(* Logix 5000 Controller export Example_PLC; controller Example_PLC 1769-L32E rev 19.11; software revision 19.01; part 2 of 6 *)

ADD_ON_INSTRUCTION AKD_Set_Decel   (* revision 2.1, ExecutePrescan, ExecuteEnableInFalse *)
// Set Drive Deceleration
// Revision note:
// Don't error if Command_Timeout preset is 0
VAR_OUTPUT
   DN : BOOL; {access Read Only, visible}   // Command Successful
   ER : BOOL; {access Read Only, visible}   // Error
END_VAR
VAR_IN_OUT
   Axis : AKD_Axis; {required}
END_VAR
VAR_INPUT
   Decel : DINT; {required}   // Acceleration
END_VAR
VAR
   Response_Bytes : SINT[8];
   OS_LoadStart : BOOL;
   Decel_Internal : DINT;   // Scaled Decel Value for Drive
   Command_Timeout : TIMER := (PRE := 100);   // Timeout Timer
   Command_Message_Type : SINT;   // Command Message Type
   Command_Axis_Number : SINT;   // Command Axis Number
   Response_Message_Type : SINT;   // Response Message Type
   Response_Axis_Number : SINT;   // Response Axis Number
   Command_Bytes : SINT[8];
   Step : SINT;
END_VAR

ROUTINE EnableInFalse   (* ladder *)
// EnableIn_False
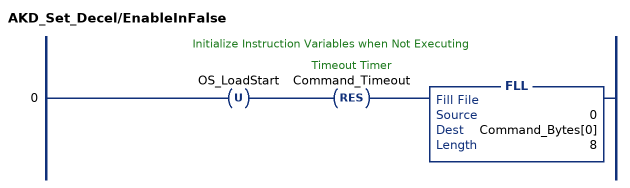
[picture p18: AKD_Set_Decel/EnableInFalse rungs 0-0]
   // Initialize Instruction Variables when Not Executing
   0: OTU(OS_LoadStart)RES(Command_Timeout)FLL(0,Command_Bytes[0],8);
END_ROUTINE

ROUTINE Logic   (* ladder *)
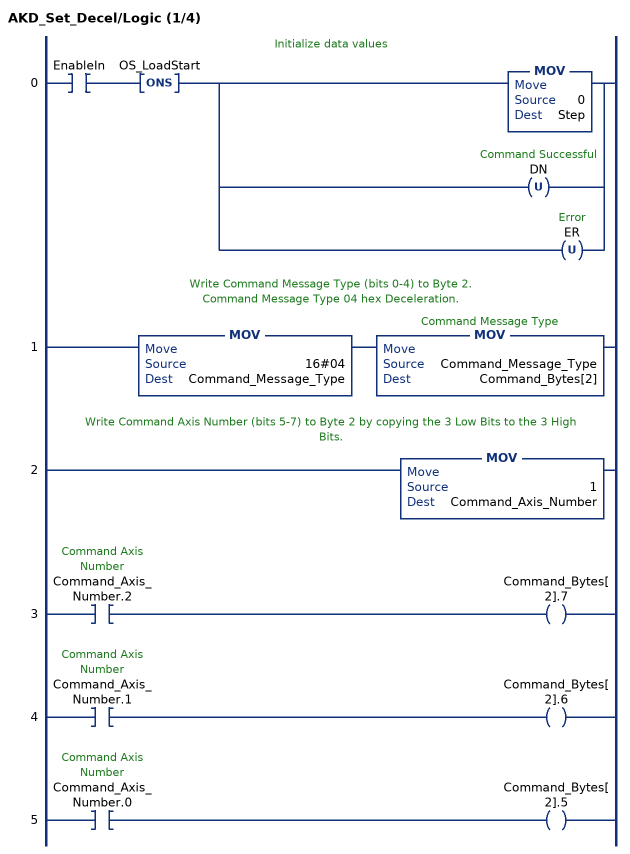
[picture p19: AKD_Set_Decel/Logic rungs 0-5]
   // Initialize data values
   0: XIC(EnableIn)ONS(OS_LoadStart)[MOV(0,Step) ,OTU(DN) ,OTU(ER) ];
   // Write Command Message Type (bits 0-4) to Byte 2.
   // Command Message Type 04 hex Deceleration.
   1: MOV(16#04,Command_Message_Type)MOV(Command_Message_Type,Command_Bytes[2]);
   // Write Command Axis Number (bits 5-7) to Byte 2 by copying the 3 Low Bits to the 3 High Bits.
   2: MOV(1,Command_Axis_Number);
   3: XIC(Command_Axis_Number.2)OTE(Command_Bytes[2].7);
   4: XIC(Command_Axis_Number.1)OTE(Command_Bytes[2].6);
   5: XIC(Command_Axis_Number.0)OTE(Command_Bytes[2].5);
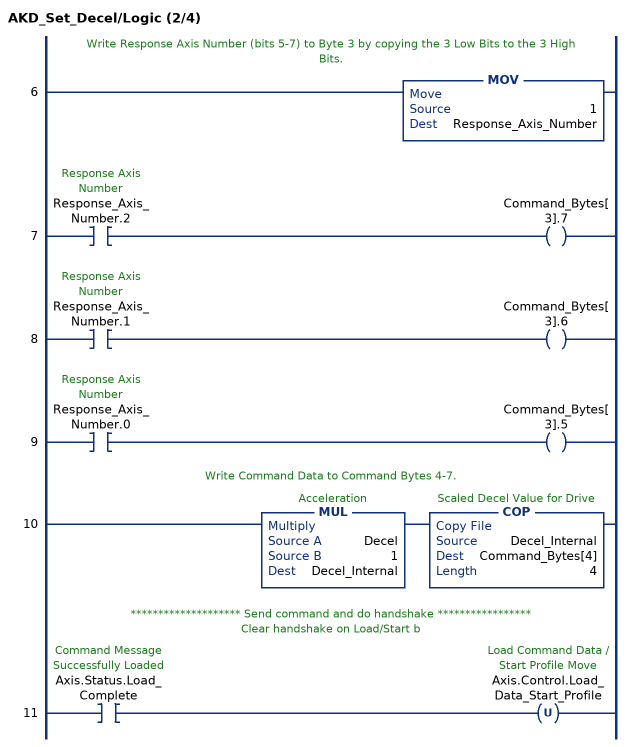
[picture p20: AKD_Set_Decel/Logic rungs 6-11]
   // Write Response Axis Number (bits 5-7) to Byte 3 by copying the 3 Low Bits to the 3 High Bits.
   6: MOV(1,Response_Axis_Number);
   7: XIC(Response_Axis_Number.2)OTE(Command_Bytes[3].7);
   8: XIC(Response_Axis_Number.1)OTE(Command_Bytes[3].6);
   9: XIC(Response_Axis_Number.0)OTE(Command_Bytes[3].5);
   // Write Command Data to Command Bytes 4-7.
   10: MUL(Decel,1,Decel_Internal)COP(Decel_Internal,Command_Bytes[4],4);
   // ******************** Send command and do handshake *****************
   // Clear handshake on Load/Start b
   11: XIC(Axis.Status.Load_Complete)OTU(Axis.Control.Load_Data_Start_Profile);
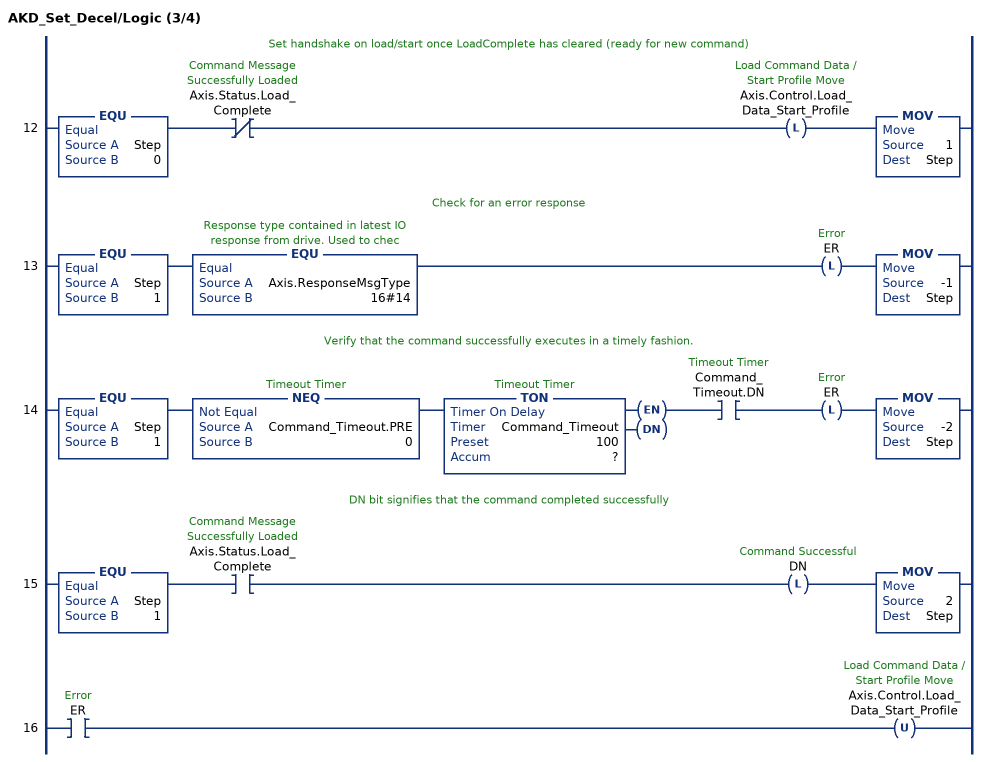
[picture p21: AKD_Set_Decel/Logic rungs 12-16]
   // Set handshake on load/start once LoadComplete has cleared (ready for new command)
   12: EQU(Step,0)XIO(Axis.Status.Load_Complete)OTL(Axis.Control.Load_Data_Start_Profile)MOV(1,Step);
   // Check for an error response
   13: EQU(Step,1)EQU(Axis.ResponseMsgType,16#14)OTL(ER)MOV(-1,Step);
   // Verify that the command successfully executes in a timely fashion.
   14: EQU(Step,1)NEQ(Command_Timeout.PRE,0)TON(Command_Timeout,?,?)XIC(Command_Timeout.DN)OTL(ER)MOV(-2,Step);
   // DN bit signifies that the command completed successfully
   15: EQU(Step,1)XIC(Axis.Status.Load_Complete)OTL(DN)MOV(2,Step);
   16: XIC(ER)OTU(Axis.Control.Load_Data_Start_Profile);
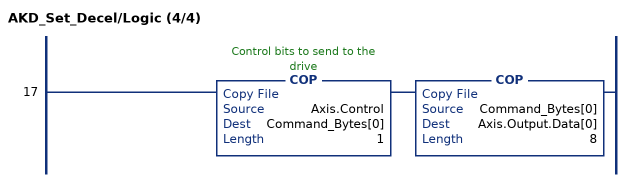
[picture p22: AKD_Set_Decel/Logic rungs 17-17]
   17: COP(Axis.Control,Command_Bytes[0],1)COP(Command_Bytes[0],Axis.Output.Data[0],8);
END_ROUTINE

ROUTINE Prescan   (* ladder *)
// Prescan
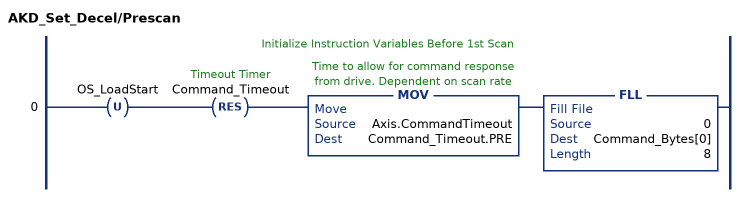
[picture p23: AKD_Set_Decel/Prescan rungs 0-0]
   // Initialize Instruction Variables Before 1st Scan
   0: OTU(OS_LoadStart)RES(Command_Timeout)MOV(Axis.CommandTimeout,Command_Timeout.PRE)FLL(0,Command_Bytes[0],8);
END_ROUTINE
END_ADD_ON_INSTRUCTION

ADD_ON_INSTRUCTION AKD_Set_Velocity   (* revision 2.1, ExecutePrescan, ExecuteEnableInFalse *)
// Set Drive Velocity
// Revision note:
// Don't error if Command_Timeout preset is 0
VAR_OUTPUT
   DN : BOOL; {access Read Only, visible}   // Command Successful
   ER : BOOL; {access Read Only, visible}   // Error
END_VAR
VAR_IN_OUT
   Axis : AKD_Axis; {required}
END_VAR
VAR_INPUT
   Velocity : DINT; {required}   // Velocity
END_VAR
VAR
   Response_Bytes : SINT[8];
   OS_LoadStart : BOOL;
   Velocity_Internal : DINT;   // Scaled Velocity Value for Drive
   Command_Timeout : TIMER := (PRE := 100);   // Timeout Timer
   Command_Message_Type : SINT;   // Command Message Type
   Command_Axis_Number : SINT;   // Command Axis Number
   Response_Message_Type : SINT;   // Response Message Type
   Response_Axis_Number : SINT;   // Response Axis Number
   Command_Bytes : SINT[8];
   Step : SINT;
END_VAR

ROUTINE EnableInFalse   (* ladder *)
// EnableIn_False
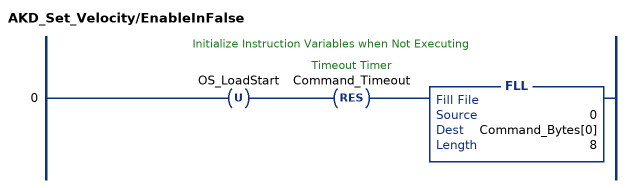
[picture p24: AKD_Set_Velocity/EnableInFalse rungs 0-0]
   // Initialize Instruction Variables when Not Executing
   0: OTU(OS_LoadStart)RES(Command_Timeout)FLL(0,Command_Bytes[0],8);
END_ROUTINE

ROUTINE Logic   (* ladder *)
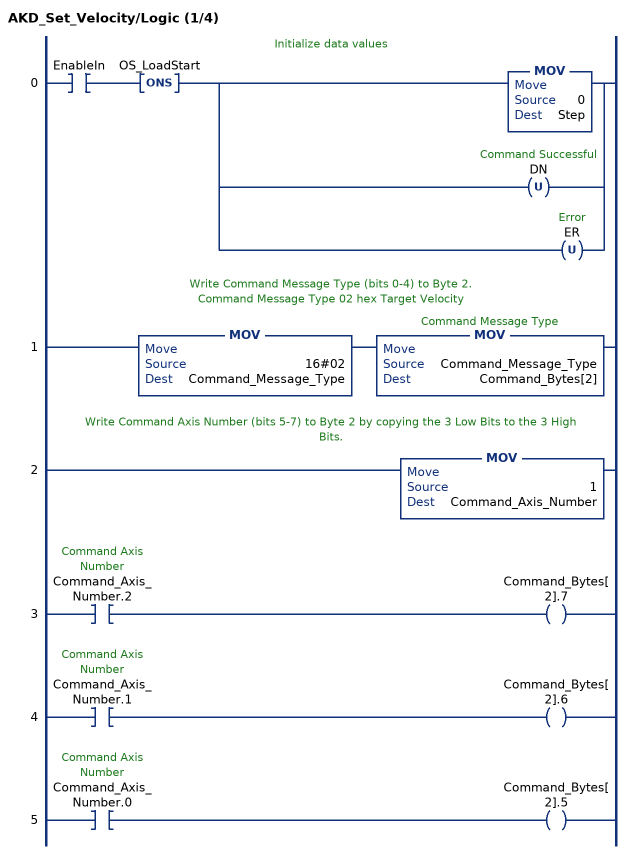
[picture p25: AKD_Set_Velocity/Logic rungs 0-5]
   // Initialize data values
   0: XIC(EnableIn)ONS(OS_LoadStart)[MOV(0,Step) ,OTU(DN) ,OTU(ER) ];
   // Write Command Message Type (bits 0-4) to Byte 2.
   // Command Message Type 02 hex Target Velocity
   1: MOV(16#02,Command_Message_Type)MOV(Command_Message_Type,Command_Bytes[2]);
   // Write Command Axis Number (bits 5-7) to Byte 2 by copying the 3 Low Bits to the 3 High Bits.
   2: MOV(1,Command_Axis_Number);
   3: XIC(Command_Axis_Number.2)OTE(Command_Bytes[2].7);
   4: XIC(Command_Axis_Number.1)OTE(Command_Bytes[2].6);
   5: XIC(Command_Axis_Number.0)OTE(Command_Bytes[2].5);
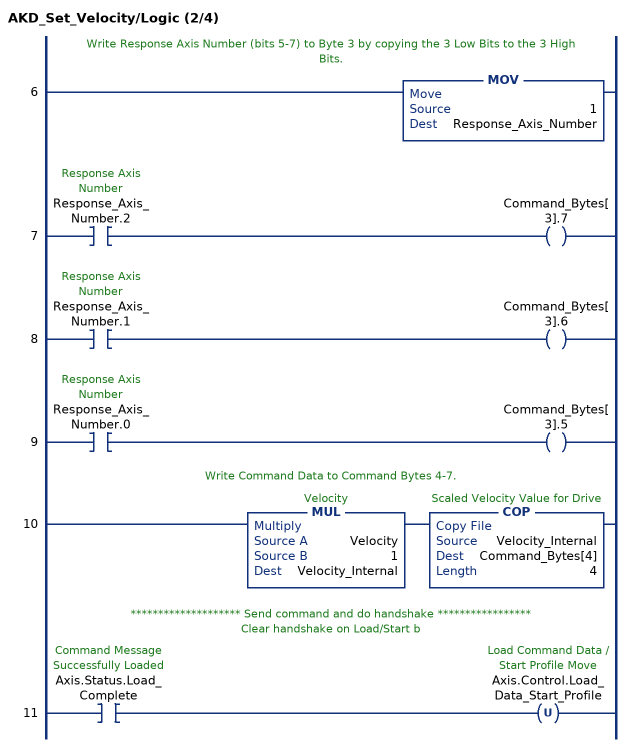
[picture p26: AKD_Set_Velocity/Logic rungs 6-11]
   // Write Response Axis Number (bits 5-7) to Byte 3 by copying the 3 Low Bits to the 3 High Bits.
   6: MOV(1,Response_Axis_Number);
   7: XIC(Response_Axis_Number.2)OTE(Command_Bytes[3].7);
   8: XIC(Response_Axis_Number.1)OTE(Command_Bytes[3].6);
   9: XIC(Response_Axis_Number.0)OTE(Command_Bytes[3].5);
   // Write Command Data to Command Bytes 4-7.
   10: MUL(Velocity,1,Velocity_Internal)COP(Velocity_Internal,Command_Bytes[4],4);
   // ******************** Send command and do handshake *****************
   // Clear handshake on Load/Start b
   11: XIC(Axis.Status.Load_Complete)OTU(Axis.Control.Load_Data_Start_Profile);
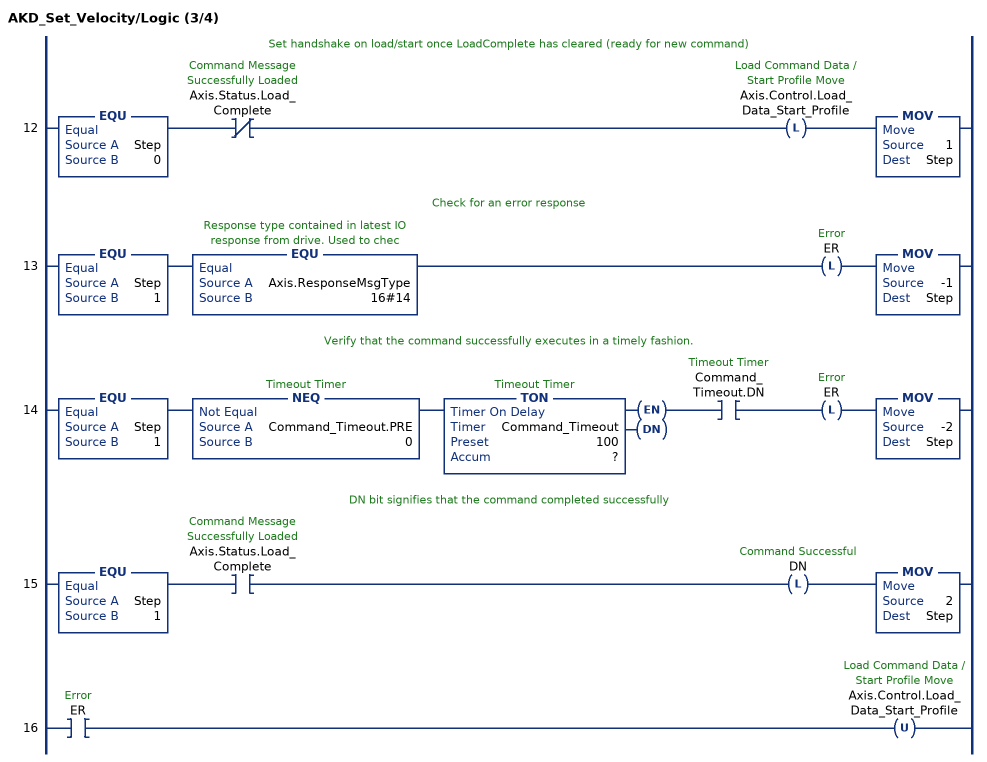
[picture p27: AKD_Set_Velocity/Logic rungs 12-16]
   // Set handshake on load/start once LoadComplete has cleared (ready for new command)
   12: EQU(Step,0)XIO(Axis.Status.Load_Complete)OTL(Axis.Control.Load_Data_Start_Profile)MOV(1,Step);
   // Check for an error response
   13: EQU(Step,1)EQU(Axis.ResponseMsgType,16#14)OTL(ER)MOV(-1,Step);
   // Verify that the command successfully executes in a timely fashion.
   14: EQU(Step,1)NEQ(Command_Timeout.PRE,0)TON(Command_Timeout,?,?)XIC(Command_Timeout.DN)OTL(ER)MOV(-2,Step);
   // DN bit signifies that the command completed successfully
   15: EQU(Step,1)XIC(Axis.Status.Load_Complete)OTL(DN)MOV(2,Step);
   16: XIC(ER)OTU(Axis.Control.Load_Data_Start_Profile);
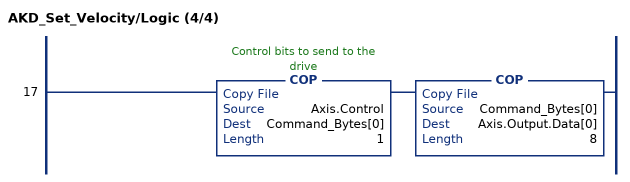
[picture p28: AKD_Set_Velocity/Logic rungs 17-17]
   17: COP(Axis.Control,Command_Bytes[0],1)COP(Command_Bytes[0],Axis.Output.Data[0],8);
END_ROUTINE

ROUTINE Prescan   (* ladder *)
// Prescan
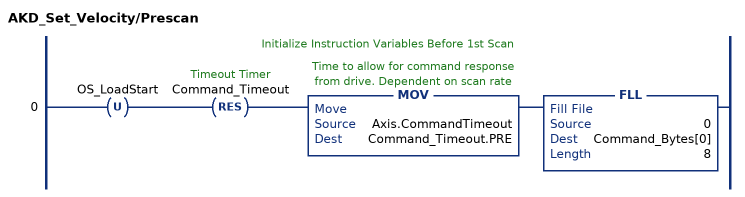
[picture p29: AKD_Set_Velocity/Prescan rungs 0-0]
   // Initialize Instruction Variables Before 1st Scan
   0: OTU(OS_LoadStart)RES(Command_Timeout)MOV(Axis.CommandTimeout,Command_Timeout.PRE)FLL(0,Command_Bytes[0],8);
END_ROUTINE
END_ADD_ON_INSTRUCTION

ADD_ON_INSTRUCTION AKD_Jog   (* revision 2.3, ExecutePrescan, ExecuteEnableInFalse *)
// Motion Axis Jog
// Revision note:
// Remove unused IP output
VAR_IN_OUT
   Axis : AKD_Axis; {required}
END_VAR
VAR_INPUT
   Accel : DINT; {required}   // Acceleration
   Decel : DINT; {required}   // Deceleration
   Direction : BOOL; {required}   // 1=Forward/Positive, 0=Reverse/Negative
   Speed : DINT; {required}   // Jog Speed
END_VAR
VAR_OUTPUT
   DN : BOOL; {access Read Only, visible}   // Command Successfully Initiated
   ER : BOOL; {access Read Only, visible}   // Error
END_VAR
VAR
   Accel_Internal : DINT;   // Scaled Accel Value for Drive
   Set_Enable : AKD_Enable;
   Set_Accel : AKD_Set_Accel;
   Set_Decel : AKD_Set_Decel;
   Set_Velocity : AKD_Set_Velocity;
   Step : SINT;   // Sequence Step Number
   Command_Axis_Number : SINT;
   Response_Axis_Number : SINT;
   OS_Start_Sequence : BOOL;
   Command_Bytes : SINT[64];
   ErrorData : SINT[8];
   Command_Timeout : TIMER := (PRE := 100);
END_VAR

ROUTINE EnableInFalse   (* ladder *)
// EnableIn_False
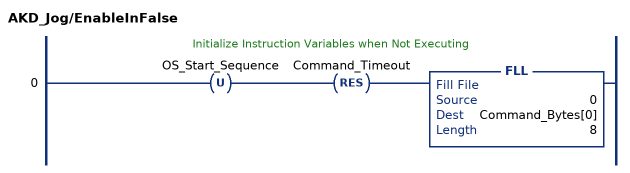
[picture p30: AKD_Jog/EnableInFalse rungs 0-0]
   // Initialize Instruction Variables when Not Executing
   0: OTU(OS_Start_Sequence)RES(Command_Timeout)FLL(0,Command_Bytes[0],8);
END_ROUTINE

ROUTINE Logic   (* ladder *)
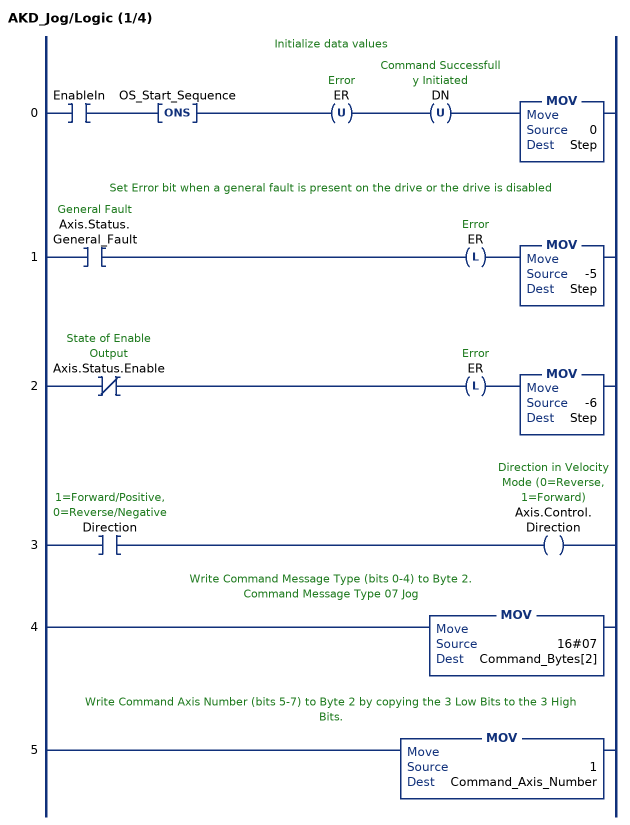
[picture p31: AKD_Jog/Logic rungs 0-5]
   // Initialize data values
   0: XIC(EnableIn)ONS(OS_Start_Sequence)OTU(ER)OTU(DN)MOV(0,Step);
   // Set Error bit when a general fault is present on the drive or the drive is disabled
   1: XIC(Axis.Status.General_Fault)OTL(ER)MOV(-5,Step);
   2: XIO(Axis.Status.Enable)OTL(ER)MOV(-6,Step);
   3: XIC(Direction)OTE(Axis.Control.Direction);
   // Write Command Message Type (bits 0-4) to Byte 2.
   // Command Message Type 07 Jog
   4: MOV(16#07,Command_Bytes[2]);
   // Write Command Axis Number (bits 5-7) to Byte 2 by copying the 3 Low Bits to the 3 High Bits.
   5: MOV(1,Command_Axis_Number);
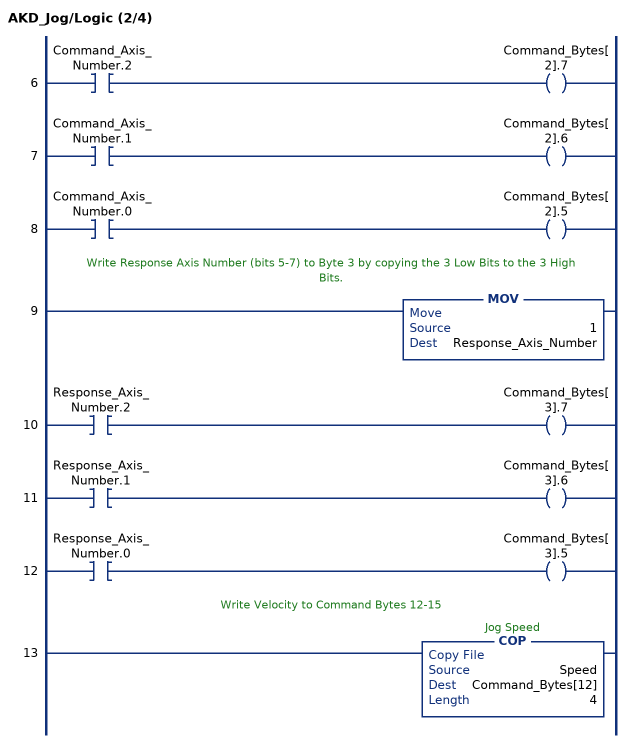
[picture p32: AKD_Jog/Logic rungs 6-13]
   6: XIC(Command_Axis_Number.2)OTE(Command_Bytes[2].7);
   7: XIC(Command_Axis_Number.1)OTE(Command_Bytes[2].6);
   8: XIC(Command_Axis_Number.0)OTE(Command_Bytes[2].5);
   // Write Response Axis Number (bits 5-7) to Byte 3 by copying the 3 Low Bits to the 3 High Bits.
   9: MOV(1,Response_Axis_Number);
   10: XIC(Response_Axis_Number.2)OTE(Command_Bytes[3].7);
   11: XIC(Response_Axis_Number.1)OTE(Command_Bytes[3].6);
   12: XIC(Response_Axis_Number.0)OTE(Command_Bytes[3].5);
   // Write Velocity to Command Bytes 12-15
   13: COP(Speed,Command_Bytes[12],4);
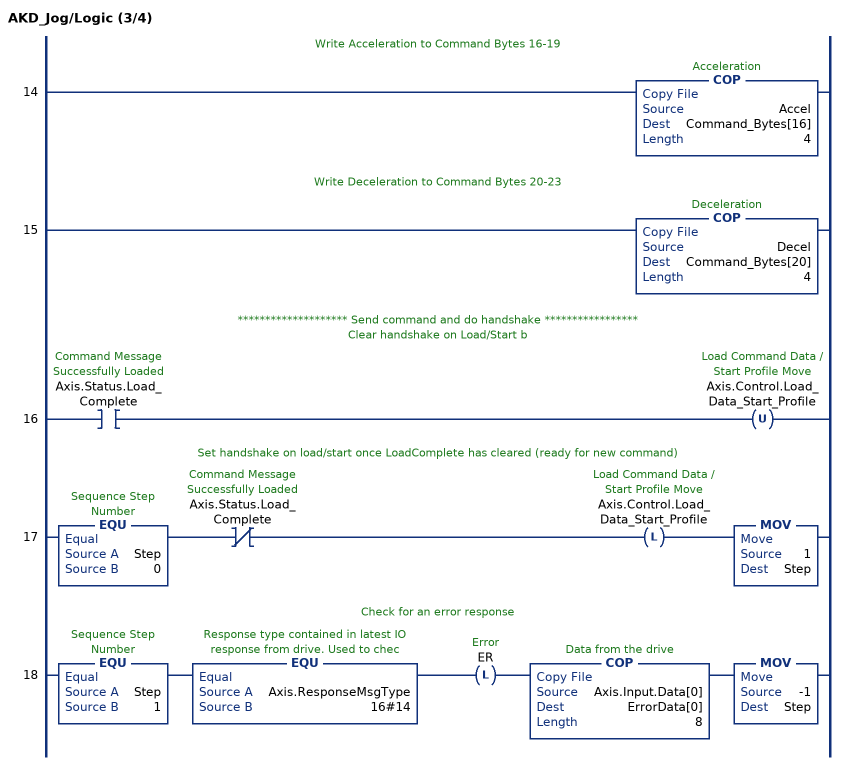
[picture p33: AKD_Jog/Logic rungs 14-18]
   // Write Acceleration to Command Bytes 16-19
   14: COP(Accel,Command_Bytes[16],4);
   // Write Deceleration to Command Bytes 20-23
   15: COP(Decel,Command_Bytes[20],4);
   // ******************** Send command and do handshake *****************
   // Clear handshake on Load/Start b
   16: XIC(Axis.Status.Load_Complete)OTU(Axis.Control.Load_Data_Start_Profile);
   // Set handshake on load/start once LoadComplete has cleared (ready for new command)
   17: EQU(Step,0)XIO(Axis.Status.Load_Complete)OTL(Axis.Control.Load_Data_Start_Profile)MOV(1,Step);
   // Check for an error response
   18: EQU(Step,1)EQU(Axis.ResponseMsgType,16#14)OTL(ER)COP(Axis.Input.Data[0],ErrorData[0],8)MOV(-1,Step);
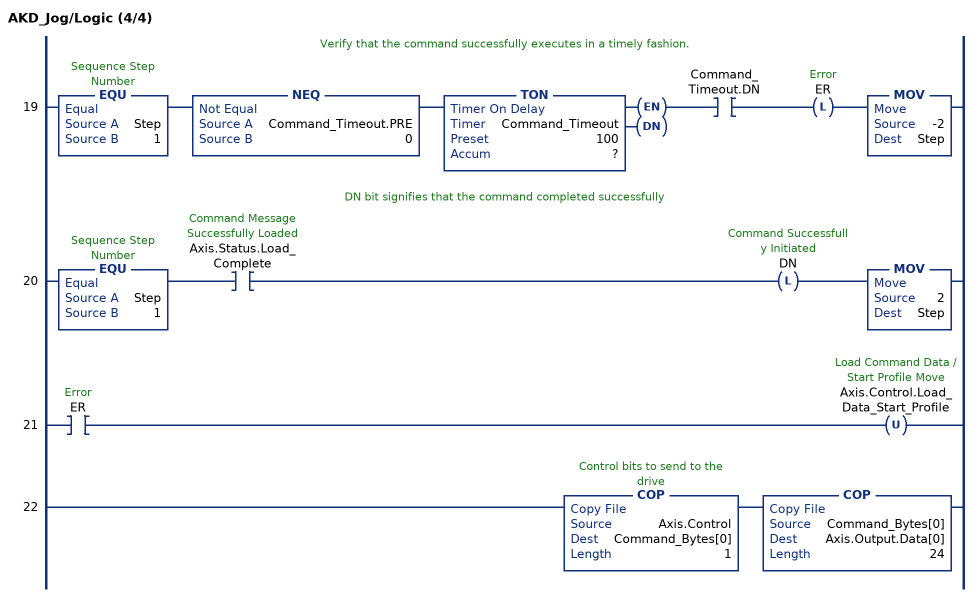
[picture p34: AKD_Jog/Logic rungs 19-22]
   // Verify that the command successfully executes in a timely fashion.
   19: EQU(Step,1)NEQ(Command_Timeout.PRE,0)TON(Command_Timeout,?,?)XIC(Command_Timeout.DN)OTL(ER)MOV(-2,Step);
   // DN bit signifies that the command completed successfully
   20: EQU(Step,1)XIC(Axis.Status.Load_Complete)OTL(DN)MOV(2,Step);
   21: XIC(ER)OTU(Axis.Control.Load_Data_Start_Profile);
   22: COP(Axis.Control,Command_Bytes[0],1)COP(Command_Bytes[0],Axis.Output.Data[0],24);
END_ROUTINE

ROUTINE Prescan   (* ladder *)
// Prescan
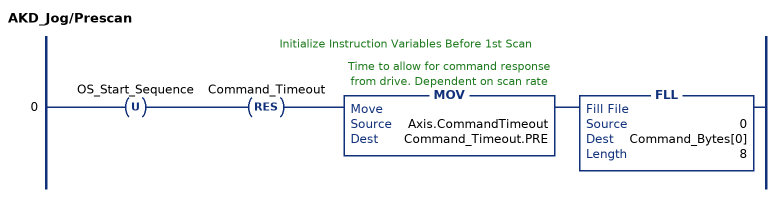
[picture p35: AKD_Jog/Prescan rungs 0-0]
   // Initialize Instruction Variables Before 1st Scan
   0: OTU(OS_Start_Sequence)RES(Command_Timeout)MOV(Axis.CommandTimeout,Command_Timeout.PRE)FLL(0,Command_Bytes[0],8);
END_ROUTINE
END_ADD_ON_INSTRUCTION
